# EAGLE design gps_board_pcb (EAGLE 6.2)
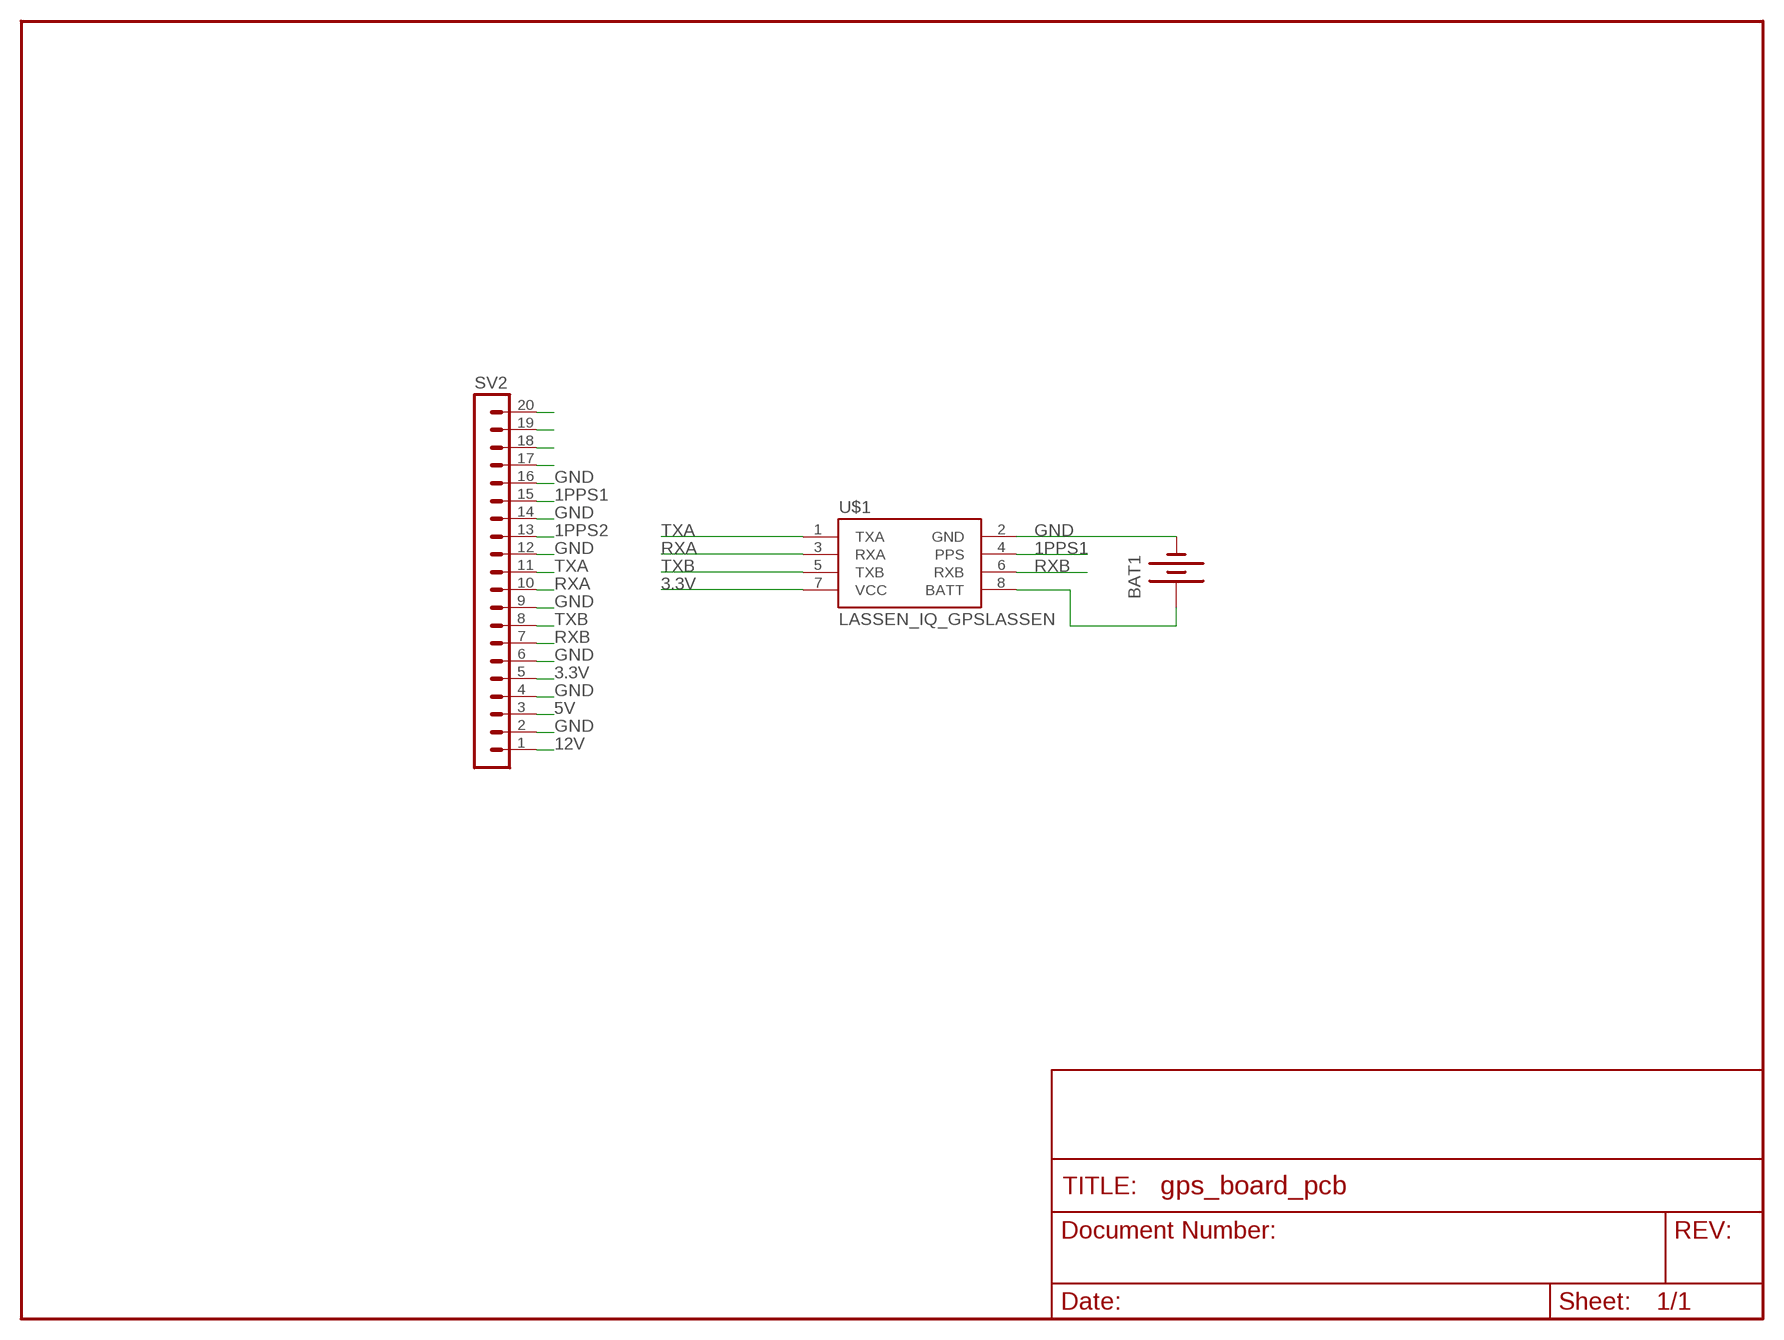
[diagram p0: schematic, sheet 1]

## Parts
BAT1  BATTERY20PTH  [BATTCOM_20MM_PTH]
SV2  MA20-1W  [MA20-1W]
U$1  LASSEN_IQ_GPSLASSEN  [LASSEN_IQ_GPS]

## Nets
1PPS1: SV2.15 U$1.4(PPS)
1PPS2: SV2.13
3.3V: SV2.5 U$1.7(VCC)
5V: SV2.3
12V: SV2.1
GND: BAT1.2(-) SV2.2 SV2.4 SV2.6 SV2.9 SV2.12 SV2.14 SV2.16 U$1.2(GND)
N$2: BAT1.1(+) U$1.8(BATT)
N$17: SV2.17
N$18: SV2.18
N$19: SV2.19
N$20: SV2.20
RXA: SV2.10 U$1.3(RXA)
RXB: SV2.7 U$1.6(RXB)
TXA: SV2.11 U$1.1(TXA)
TXB: SV2.8 U$1.5(TXB)

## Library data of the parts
BAT1 = SparkFun:BATTERY: Battery Holders
SV2 = con-lstb:MA20-1W: PIN HEADER; OC_FARNELL: unknown; OC_NEWARK: unknown
U$1 = SparkFun:LASSEN_IQ_GPS: Lassen iq 12-Channel GPS receiver. Schematic and footprint production proven. Spark Fun Electronics SKU : GPS-00163. Surface mount mating connector : GPS-00170

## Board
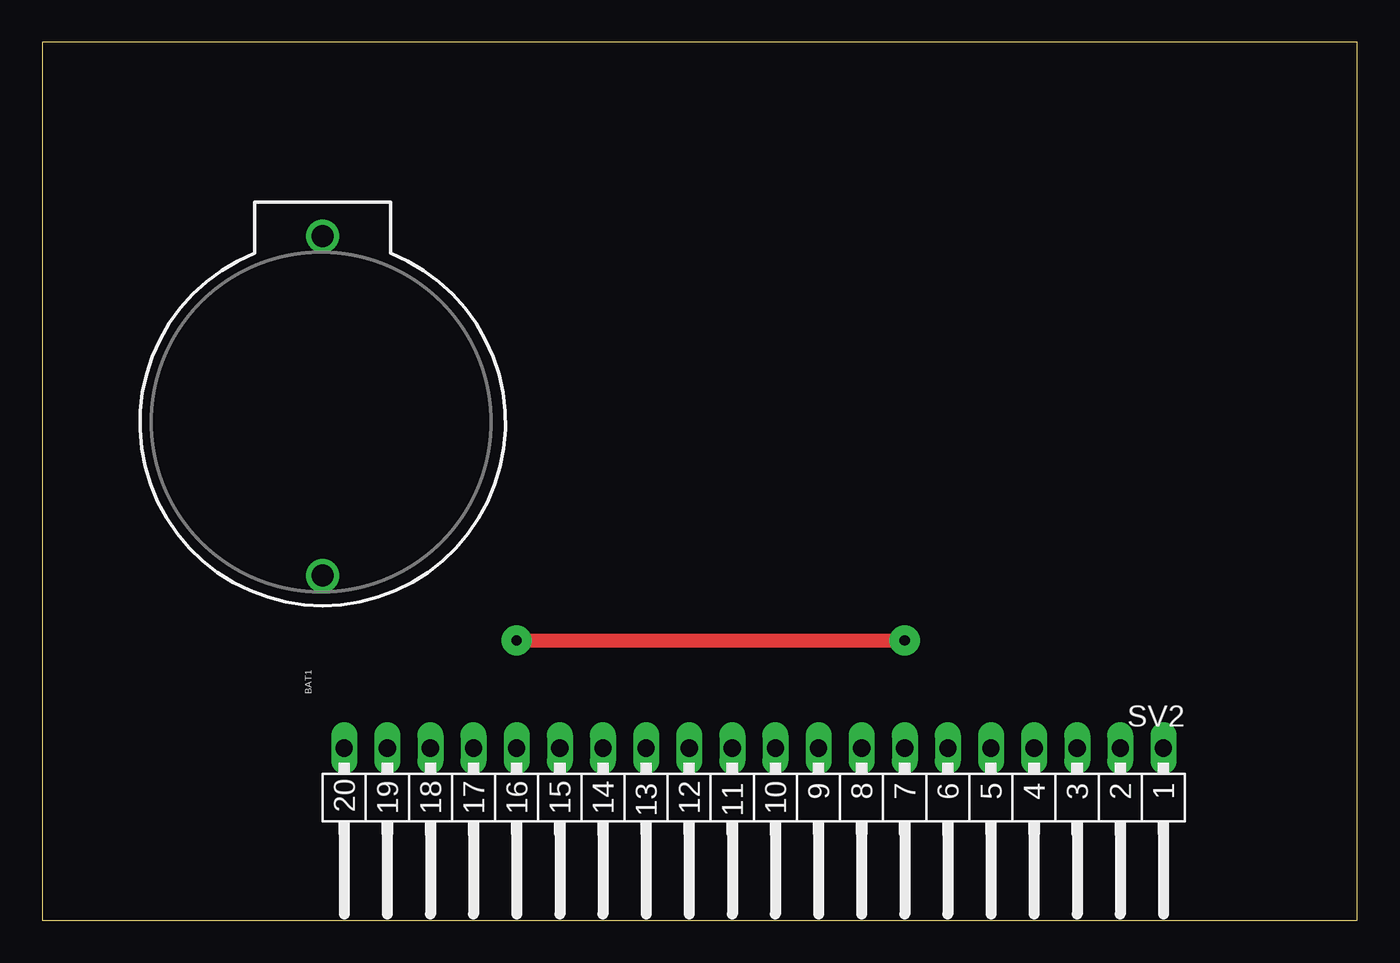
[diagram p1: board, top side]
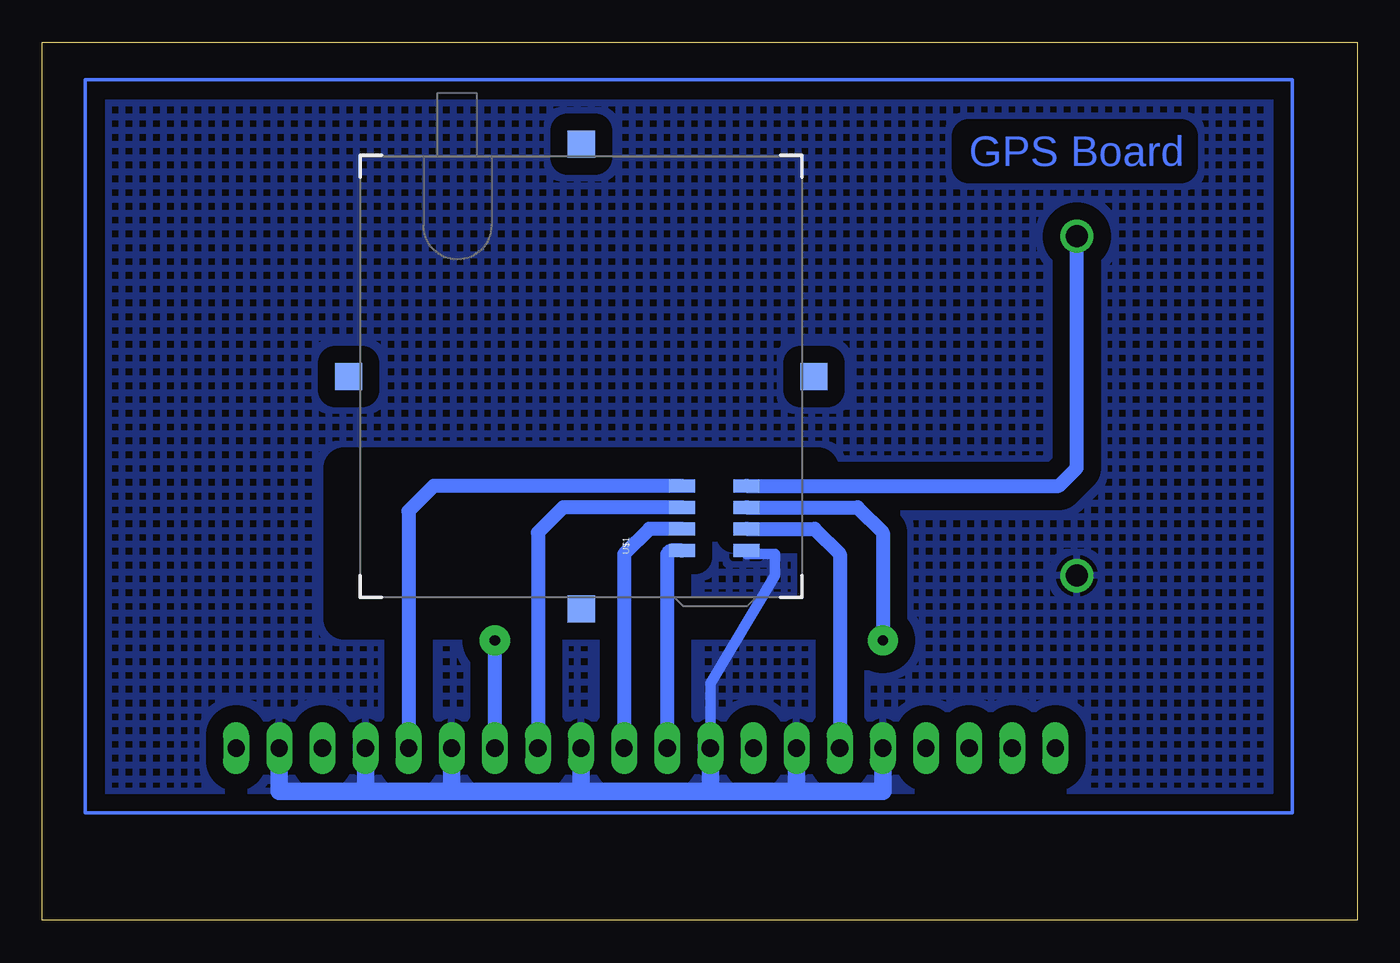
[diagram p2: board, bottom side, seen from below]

Size 77.45 x 51.74 mm. Coordinates in mm from the lower left corner, seen from the top.
Outline: 0,0 77.45,0 77.45,51.74 0,51.74 0,0
Copper layers (1*16): Top 0.035mm / dielectric 1.5mm / Bottom 0.035mm
Design rules: minimum track width 10mil, minimum drill 24mil, track to track 8mil, track to pad 8mil, pad to pad 8mil, via to via 8mil, smd to smd 8mil, copper to edge 40mil, drill to drill 8mil, minimum pad ring 10mil, minimum via ring 8mil, stop-mask expansion 4mil, vias tented up to drill 0mil, thermal gap 10mil
bRestrict: 4 lines

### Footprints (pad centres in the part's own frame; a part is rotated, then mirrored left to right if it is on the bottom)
BATTCOM_20MM_PTH = drill 1.3: 1 20,0; 2 0,0
MA20-1W = drill 1.016 long: 1 -24.13,0; 2 -21.59,0; 3 -19.05,0; 4 -16.51,0; 5 -13.97,0; 6 -11.43,0; 7 -8.89,0; 8 -6.35,0; 9 -3.81,0; 10 -1.27,0; 11 1.27,0; 12 3.81,0; 13 6.35,0; 14 8.89,0; 15 11.43,0; 16 13.97,0; 17 16.51,0; 18 19.05,0; 19 21.59,0; 20 24.13,0
LASSEN_IQ_GPS = smd 0.762 x 1.524: 1 2.752,7.076; 2 2.752,3.266; 3 4.022,7.076; 4 4.022,3.266; 5 5.292,7.076; 6 5.292,3.266; 7 6.562,7.076; 8 6.562,3.266 | smd 1.6 x 1.6: GND1 -0.7,13; GND2 13,26.7; GND3 26.7,13; GND4 13,-0.7

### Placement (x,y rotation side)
BAT1  16.51,20.32 90 top
SV2  41.91,10.16 180 top
U$1  32.7,19.05 90 bottom

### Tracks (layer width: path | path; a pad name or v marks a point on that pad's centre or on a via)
1PPS1
  Bottom 0.813: U$1.4 31.96,23.07 30.48,21.59 SV2.15
3.3V
  Bottom 0.813: U$1.7 54.4,25.61 55.88,24.13 SV2.5
GND
  Bottom 0.61: SV2.12 38.1,13.97 34.29,20.32 34.29,21.59 35.97,21.59 U$1.2
  Bottom 1.016: SV2.2 63.5,7.62 58.42,7.62 | SV2.4 58.42,7.62 | 58.42,7.62 53.34,7.62 | SV2.6 53.34,7.62 | 53.34,7.62 45.72,7.62 | SV2.9 45.72,7.62 | 45.72,7.62 38.1,7.62 | SV2.12 38.1,7.62 | 38.1,7.62 33.02,7.62 | SV2.14 33.02,7.62 | 33.02,7.62 27.94,7.62 SV2.16
  pour Bottom (isolate 1.016, hatched): 5.08,48.26 73.66,48.26 73.66,7.62 5.08,7.62
N$2
  Bottom 0.813: U$1.8 17.57,25.61 16.51,26.67 BAT1.1
N$5
  Bottom 0.2: 74.93,6.35 3.81,6.35 3.81,49.53 74.93,49.53 74.93,6.35
RXA
  Bottom 0.813: U$1.3 41.7,23.07 43.18,21.59 SV2.10
RXB  (via drill 0.6, 0.6 pad 1.78)
  Top 0.813: v27.94,16.51 v50.8,16.51
  Bottom 0.813: U$1.6 29.42,24.34 27.94,22.86 v27.94,16.51 | v50.8,16.51 SV2.7
TXA
  Bottom 0.813: U$1.1 40.43,21.8 40.64,21.59 SV2.11
TXB
  Bottom 0.813: U$1.5 46.78,24.34 48.26,22.86 SV2.8

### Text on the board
Bottom: GPS Board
